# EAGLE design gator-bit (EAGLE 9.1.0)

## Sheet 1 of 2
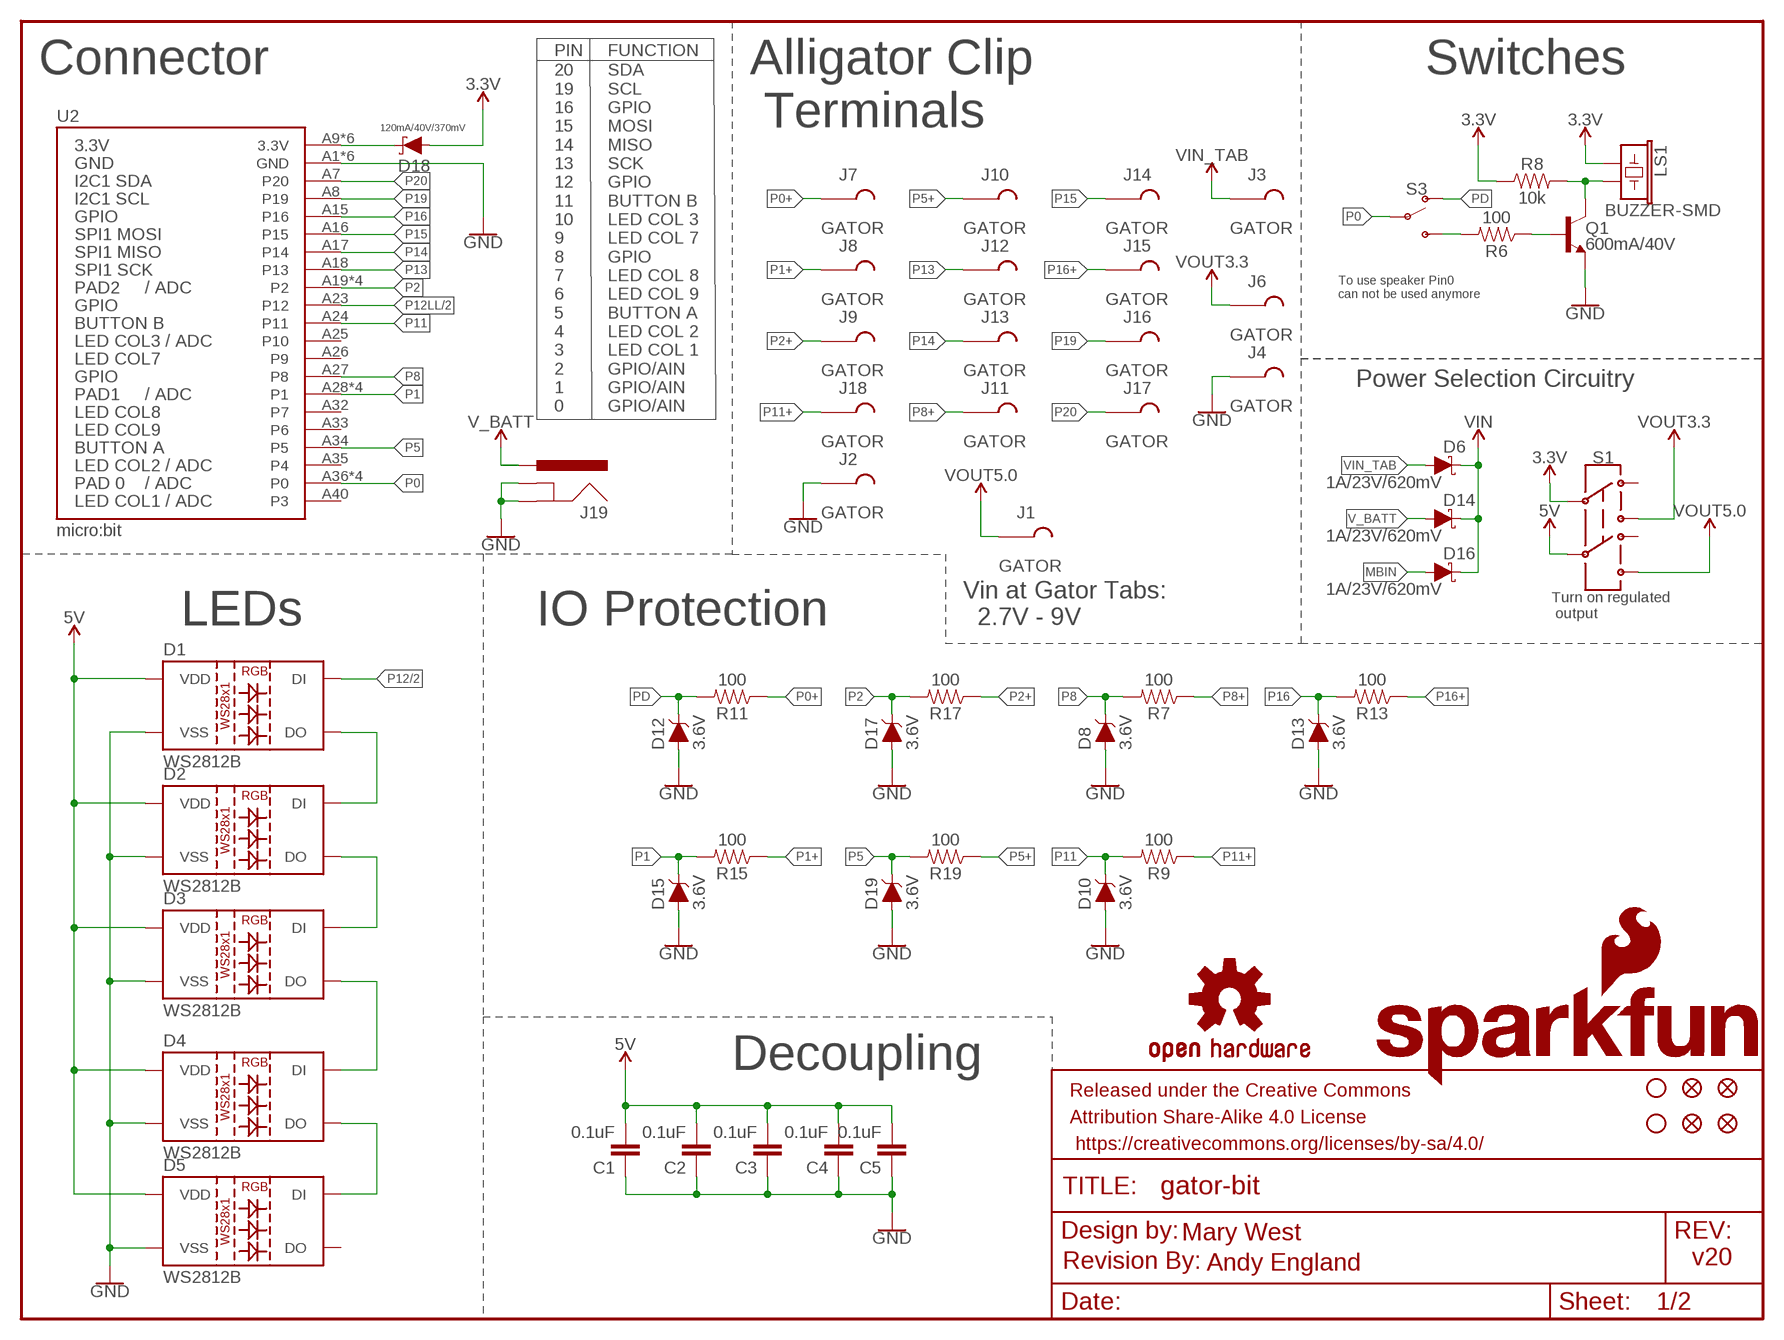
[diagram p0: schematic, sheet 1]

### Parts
C1  0.1uF  0.1UF-0603-25V-(+80/-20%)  [0603]
C2  0.1uF  0.1UF-0603-25V-(+80/-20%)  [0603]
C3  0.1uF  0.1UF-0603-25V-(+80/-20%)  [0603]
C4  0.1uF  0.1UF-0603-25V-(+80/-20%)  [0603]
C5  0.1uF  0.1UF-0603-25V-(+80/-20%)  [0603]
D1  WS2812B  [WS2812B]
D2  WS2812B  [WS2812B]
D3  WS2812B  [WS2812B]
D4  WS2812B  [WS2812B]
D5  WS2812B  [WS2812B]
D6  1A/23V/620mV  DIODE-SCHOTTKY-BAT20J  [SOD-323]
D8  3.6V  DIODE-ZENER-BZT52C3V6S  [SOD-323]
D10  3.6V  DIODE-ZENER-BZT52C3V6S  [SOD-323]
D12  3.6V  DIODE-ZENER-BZT52C3V6S  [SOD-323]
D13  3.6V  DIODE-ZENER-BZT52C3V6S  [SOD-323]
D14  1A/23V/620mV  DIODE-SCHOTTKY-BAT20J  [SOD-323]
D15  3.6V  DIODE-ZENER-BZT52C3V6S  [SOD-323]
D16  1A/23V/620mV  DIODE-SCHOTTKY-BAT20J  [SOD-323]
D17  3.6V  DIODE-ZENER-BZT52C3V6S  [SOD-323]
D18  120mA/40V/370mV  DIODE-SCHOTTKY-RB751S40  [SOD-523]
D19  3.6V  DIODE-ZENER-BZT52C3V6S  [SOD-323]
FD1  FIDUCIAL1X2  [FIDUCIAL-1X2]
FD2  FIDUCIAL1X2  [FIDUCIAL-1X2]
FD3  FIDUCIAL1X2  [FIDUCIAL-1X2]
FD4  FIDUCIAL1X2  [FIDUCIAL-1X2]
FRAME1  FRAME-LETTER  [CREATIVE_COMMONS]
H1  STAND-OFF  [STAND-OFF]
H2  STAND-OFF  [STAND-OFF]
J1  GATOR  [GATOR]
J2  GATOR  [GATOR]
J3  GATOR  [GATOR]
J4  GATOR  [GATOR]
J6  GATOR  [GATOR]
J7  GATOR  [GATOR]
J8  GATOR  [GATOR]
J9  GATOR  [GATOR]
J10  GATOR  [GATOR]
J11  GATOR  [GATOR]
J12  GATOR  [GATOR]
J13  GATOR  [GATOR]
J14  GATOR  [GATOR]
J15  GATOR  [GATOR]
J16  GATOR  [GATOR]
J17  GATOR  [GATOR]
J18  GATOR  [GATOR]
J19  POWER_JACKPTH_LOCK  [POWER_JACK_PTH_LOCK]
LOGO1  SFE_LOGO_NAME_FLAME.3_INCH  [SFE_LOGO_NAME_FLAME_.3]
LOGO2  OSHW-LOGOM  [OSHW-LOGO-M]
LOGO3  REVISION  [REVISION]
LS1  BUZZER-SMD  [BUZZER-CCV]
Q1  600mA/40V  TRANS_NPN-MMBT2222AL  [SOT23-3]
R6  100  100OHM-0603-1/10W-1%  [0603]
R7  100  100OHM-0603-1/10W-1%  [0603]
R8  10k  10KOHM-0603-1/10W-1%  [0603]
R9  100  100OHM-0603-1/10W-1%  [0603]
R11  100  100OHM-0603-1/10W-1%  [0603]
R13  100  100OHM-0603-1/10W-1%  [0603]
R15  100  100OHM-0603-1/10W-1%  [0603]
R17  100  100OHM-0603-1/10W-1%  [0603]
R19  100  100OHM-0603-1/10W-1%  [0603]
S1  SWITCH-DPDT-SMD-AYZ0202  [SWITCH_DPDT_SMD_AYZ0202]
S3  SWITCH-SPDT-SMD-AYZ0202  [SWITCH_DPDT_SMD_AYZ0202]
U2  micro:bit  MICRO:BITLEDS_UP  [MICRO:BIT_RA_PTH]

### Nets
3.3V: D18.A LS1.+ R8.1 S1.2 ; also sheet 2
5V: C1.2 C2.2 C3.2 C4.2 C5.2 D1.1(VDD) D2.1(VDD) D3.1(VDD) D4.1(VDD) D5.1(VDD) S1.5 ; also sheet 2
GND: C1.1 C2.1 C3.1 C4.1 C5.1 D1.3(VSS) D2.3(VSS) D3.3(VSS) D4.3(VSS) D5.3(VSS) D8.A D10.A D12.A D13.A D15.A D17.A D19.A J2.P$1 J2.P$2 J4.P$1 J4.P$2 J19.GND J19.GNDBREAK Q1.2(E) U2.A1(GND) U2.A2(GND) U2.A3(GND) U2.A4(GND) U2.A5(GND) U2.A6(GND) ; also sheet 2
MBIN: D16.A D18.C U2.A9(3.3V) U2.A10(3.3V) U2.A11(3.3V) U2.A12(3.3V) U2.A13(3.3V) U2.A14(3.3V)
N$3: LS1.- Q1.3(C) R8.2
N$4: D1.2(DO) D2.4(DI)
N$5: D2.2(DO) D3.4(DI)
N$6: D3.2(DO) D4.4(DI)
N$7: D4.2(DO) D5.4(DI)
N$20: R6.2 S3.3(S)
N$25: Q1.1(B) R6.1
P0: S3.2(P) U2.A36(P0) U2.A37(P0) U2.A38(P0) U2.A39(P0)
P0+: J7.P$1 J7.P$2 R11.1
P1: D15.C R15.2 U2.A28(P1) U2.A29(P1) U2.A30(P1) U2.A31(P1)
P1+: J8.P$1 J8.P$2 R15.1
P2: D17.C R17.2 U2.A19(P2) U2.A20(P2) U2.A21(P2) U2.A22(P2)
P2+: J9.P$1 J9.P$2 R17.1
P5: D19.C R19.2 U2.A34(P5)
P5+: J10.P$1 J10.P$2 R19.1
P8: D8.C R7.2 U2.A27(P8)
P8+: J11.P$1 J11.P$2 R7.1
P11: D10.C R9.2 U2.A24(P11)
P11+: J18.P$1 J18.P$2 R9.1
P12: D1.4(DI) ; also sheet 2
P12LL: U2.A23(P12) ; also sheet 2
P13: J12.P$1 J12.P$2 U2.A18(P13)
P14: J13.P$1 J13.P$2 U2.A17(P14)
P15: J14.P$1 J14.P$2 U2.A16(P15)
P16: D13.C R13.2 U2.A15(P16)
P16+: J15.P$1 J15.P$2 R13.1
P19: J16.P$1 J16.P$2 U2.A8(P19)
P20: J17.P$1 J17.P$2 U2.A7(P20)
PD: D12.C R11.2 S3.1(O)
V_BATT: D14.A J19.PWR
VIN: D6.C D14.C D16.C ; also sheet 2
VIN_TAB: D6.A J3.P$1 J3.P$2
VOUT3.3: J6.P$1 J6.P$2 S1.3 ; also sheet 2
VOUT5.0: J1.P$1 J1.P$2 S1.6 ; also sheet 2
Unconnected: D5.2(DO) S1.1 S1.4 U2.A25(P10) U2.A26(P9) U2.A32(P7) U2.A33(P6) U2.A35(P4) U2.A40(P3)

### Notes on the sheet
- PIN | FUNCTION
- Connector | Switches
- Alligator Clip
   Terminals
- To use speaker Pin0 
  can not be used anymore
- Power Selection Circuitry
- 20
  19
  16
  15
  14
  13
  12
  11
  10
  9
  8
  7
  6
  5
  4
  3
  2
  1
  0
- SDA
  SCL
  GPIO
  MOSI
  MISO
  SCK
  GPIO
  BUTTON B
  LED COL 3
  LED COL 7
  GPIO
  LED COL 8
  LED COL 9
  BUTTON A
  LED COL 2
  LED COL 1
  GPIO/AIN
  GPIO/AIN
  GPIO/AIN
- Turn on regulated
   output
- LEDs | IO Protection
- Vin at Gator Tabs:
    2.7V - 9V
- Decoupling
- Mary West
- Andy England | v20

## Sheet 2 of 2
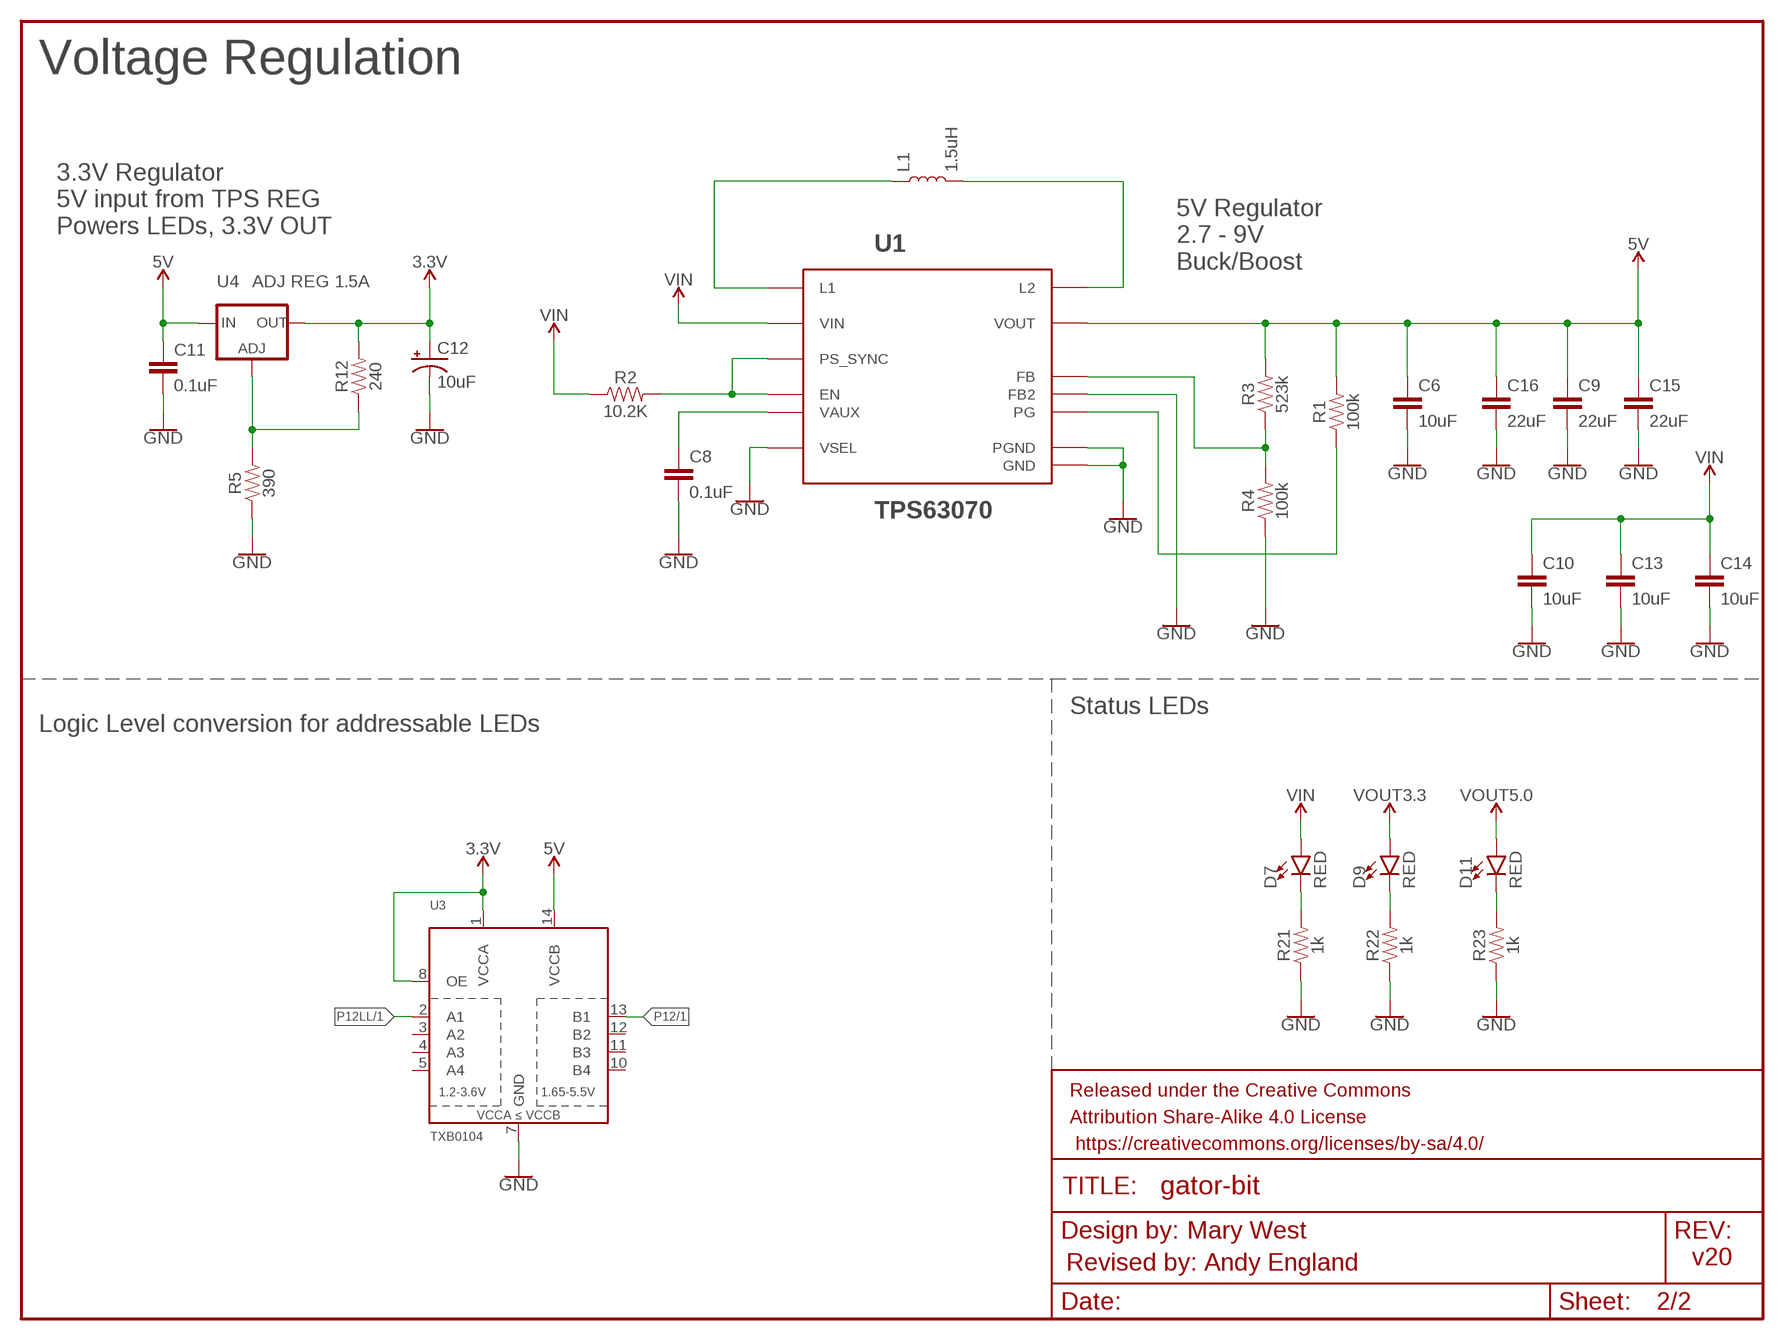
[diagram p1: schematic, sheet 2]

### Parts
C6  10uF  10UF-0603-6.3V-20%  [0603]
C8  0.1uF  0.1UF-0603-25V-(+80/-20%)  [0603]
C9  22uF  22UF-0805-6.3V-20%  [0805]
C10  10uF  10UF-0805-10V-10%  [0805]
C11  0.1uF  0.1UF-0603-25V-(+80/-20%)  [0603]
C12  10uF  10UF-POLAR-EIA3216-16V-10%(TANT)  [EIA3216]
C13  10uF  10UF-0805-10V-10%  [0805]
C14  10uF  10UF-0603-6.3V-20%  [0603]
C15  22uF  22UF-0805-6.3V-20%  [0805]
C16  22uF  22UF-0805-6.3V-20%  [0805]
D7  RED  LED-RED0603  [LED-0603]
D9  RED  LED-RED0603  [LED-0603]
D11  RED  LED-RED0603  [LED-0603]
FRAME3  FRAME-LETTER  [CREATIVE_COMMONS]
L1  1.5uH  INDUCTOR-XFL40201.5UH  [XFL4020]
R1  100k  100KOHM-0603-1/10W-1%  [0603]
R2  10.2K  10.2KOHM  [0603]
R3  523k  523KOHMOHMS-0603-1/10W-1%  [0603]
R4  100k  100KOHM-0603-1/10W-1%  [0603]
R5  390  390OHM-0603-1/10W-1%  [0603]
R12  240  240OHM-0603-1/10W-1%  [0603]
R21  1k  1KOHM-0603-1/10W-1%  [0603]
R22  1k  1KOHM-0603-1/10W-1%  [0603]
R23  1k  1KOHM-0603-1/10W-1%  [0603]
U1  TPS63070  TPS63070RNM  [TPS63070RNM]
U3  TXB0104  TXB0104PWR  [TSSOP14]
U4  ADJ REG 1.5A  GATORBIT_LM317  [SOT223]

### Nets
3.3V: C12.+ R12.2 U3.1(VCCA) U3.8(OE) U4.2(OUT) U4.4(OUT) ; also sheet 1
5V: C6.1 C9.1 C11.1 C15.1 C16.1 R1.2 R3.2 U1.P$7(VOUT) U3.14(VCCB) U4.3(IN) ; also sheet 1
GND: C6.2 C8.2 C9.2 C10.2 C11.2 C12.- C13.2 C14.2 C15.2 C16.2 R4.1 R5.1 R21.1 R22.1 R23.1 U1.P$4(GND) U1.P$6(FB2) U1.P$10(PGND) U1.P$15(VSEL) U3.7(GND) ; also sheet 1
N$2: L1.P$1 U1.P$11(L1)
N$8: L1.P$2 U1.P$9(L2)
N$9: D7.C R21.2
N$11: R3.1 R4.2 U1.P$5(FB)
N$12: C8.1 U1.P$3(VAUX)
N$13: R2.2 U1.P$1(PS_SYNC) U1.P$14(EN)
N$14: R1.1 U1.P$2(PG)
N$16: R5.2 R12.1 U4.1(ADJ)
N$23: D9.C R22.2
N$24: D11.C R23.2
P12: U3.13(B1) ; also sheet 1
P12LL: U3.2(A1) ; also sheet 1
VIN: C10.1 C13.1 C14.1 D7.A R2.1 U1.P$12(VIN) ; also sheet 1
VOUT3.3: D9.A ; also sheet 1
VOUT5.0: D11.A ; also sheet 1
Unconnected: U3.3(A2) U3.4(A3) U3.5(A4) U3.10(B4) U3.11(B3) U3.12(B2)

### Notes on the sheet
- Voltage Regulation
- 3.3V Regulator
  5V input from TPS REG
  Powers LEDs, 3.3V OUT
- 5V Regulator
  2.7 - 9V
  Buck/Boost
- Status LEDs
- Logic Level conversion for addressable LEDs
- Mary West
- Revised by: Andy England | v20

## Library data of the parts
C1-C5 C8 C11 = SparkFun-Capacitors:0.1UF: 0.1µF ceramic capacitors; PROD_ID: CAP-00810
C6 C14 = SparkFun-Capacitors:10UF: 10.0µF ceramic capacitors; PROD_ID: CAP-11015
C9 C15 C16 = SparkFun-Capacitors:22UF: 22µF ceramic capacitors; PROD_ID: CAP-08402
C10 C13 = SparkFun-Capacitors:10UF: 10.0µF ceramic capacitors; PROD_ID: CAP-11330
C12 = SparkFun-Capacitors:10UF-POLAR: 10.0µF polarized capacitors; PROD_ID: CAP-00811
D1-D5 = SparkFun-LED:WS2812B: WS2812B SMD addressable RGB LED 5x5mm SMD LED with built-in controller IC. Color: Red/Green/Blue mC Rating: RGB: 390, 660, 180 mcd Forward Voltage: RGB: 2.0, 3.0, 3.0 V Packages:WS2812B SparkFun Products: Blynk Board - ESP8266; PROD_ID: DIO-12503
D6 D14 D16 = SparkFun-DiscreteSemi:DIODE-SCHOTTKY: Schottky diode; PROD_ID: DIO-11623
D7 D9 D11 = SparkFun-LED:LED-RED: Red SMD LED; PROD_ID: DIO-00819
D8 D10 D12 D13 D15 D17 D19 = SparkFun-DiscreteSemi:DIODE-ZENER: Zener Diode; PROD_ID: DIO-08199
D18 = SparkFun-DiscreteSemi:DIODE-SCHOTTKY: Schottky diode; PROD_ID: DIO-11018
FD1-FD4 = SparkFun-Aesthetics:FIDUCIAL: Fiducial Alignment Points
FRAME1 FRAME3 = SparkFun-Aesthetics:FRAME-LETTER: Schematic Frame - Letter
H1 H2 = SparkFun-Hardware:STAND-OFF: Stand Off
J1-J4 J6-J18 = TAB:GATOR
J19 = SparkFun-Connectors:POWER_JACK: Power Jack Connector This is the standard 5.5mm barrel jack for power. The PTH is the most common, proven, reliable, footprint. The Slot footprint only works if the mill layer is transmitted to the PCB fab house so be warned. Here are the connectors we sell at SparkFun: DC Barrel Power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; PROD_ID: CONN-08197; SF_ID: PRT-00119
L1 = SparkFun-Coils:INDUCTOR-XFL4020; PROD_ID: INDUC-13855
LOGO1 = SparkFun-Aesthetics:SFE_LOGO_NAME_FLAME: SparkFun Font Logo w/ Flame
LOGO2 = SparkFun-Aesthetics:OSHW-LOGO: Open-Source Hardware (OSHW) Logo
LOGO3 = SparkFun-Aesthetics:REVISION: "Revision By" Text
LS1 = SparkFun-Electromechanical:BUZZER: Buzzer; PROD_ID: COMP-08568
Q1 = SparkFun-DiscreteSemi:TRANS_NPN: NPN transistor Current controlled devices typically used to amplify current or used as a switch. BC547 - COM-08928 (TO-92 45V 100mA) (1.Collector 2.Base 3.Emitter) 2N3904 - COM-00521 (TO-92 40V 200mA) (1.Emitter 2.Base 3.Collector) P2N2222A - COM-12852 (TO-92 40V 600mA) (1.Collector 2.Base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; PROD_ID: TRANS-08049
R1 R4 = SparkFun-Resistors:100KOHM: 100kΩ resistor; PROD_ID: RES-07828
R2 = SparkFun-Resistors:10.2KOHM: https://www.digikey.com/product-detail/en/yageo/RC0603FR-0710K2L/311-10.2KHRTR-ND/726883; PROD_ID: RES-13856
R3 = SparkFun-Resistors:523KOHM; PROD_ID: RES-13864
R5 = SparkFun-Resistors:390OHM: 390Ω resistor; PROD_ID: RES-07864
R6 R7 R9 R11 R13 R15 R17 R19 = SparkFun-Resistors:100OHM: 100Ω resistor; PROD_ID: RES-07863
R8 = SparkFun-Resistors:10KOHM: 10kΩ resistor; PROD_ID: RES-00824
R12 = SparkFun-Resistors:240OHM: 240Ω resistor; PROD_ID: RES-07849
R21-R23 = SparkFun-Resistors:1KOHM: 1kΩ resistor; PROD_ID: RES-07856
S1 = SparkFun-Switches:SWITCH-DPDT: Double-Pole, Double-Throw (DPDT) Switch Double-pole, double-throw switches. Variant Overview PTH-GPI-152-3013 Used on SparkFun Geiger Counter SMD-AY0202 Surface Mount DPDT Switch (COM-00597) Used on e.g. LilyPad Arduino USB - ATmega32U4 Board; PROD_ID: SWCH-08179; SF_SKU: COM-00597
S3 = SparkFun-Switches:SWITCH-SPDT: Single Pole, Double Throw (SPDT) Switch Single-pole, double-throw (SPDT) switch. Variant Overview SMD-AYZ0202 Surface Mount DPDT Switch (COM-00597) Used on e.g. LilyPad Arduino USB - ATmega32U4 Board PTH-11.6X4.0MM SPDT Mini Power Switch (COM-00102) Used on e.g. SparkFun Simon Says - Through-Hole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; PROD_ID: SWCH-08179; SF_ID: COM-00597
U1 = SparkFun-IC-Power:TPS63070RNM: The TPS6307x is a high efficiency, low quiescent current buck-boost converter suitable for applications where the input voltage can be higher or lower than the output voltage. Output currents can go as high as 2 A in boost mode and in buck mode. The buck-boost converter is based on a fixed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; PROD_ID: IC-13858
U2 = Micro_Bit_Parts:MICRO:BIT: BBC MICRO_BIT with 5x5 LED array facing the direction noted in the variant. "UP" means away from the host board, "Down" means facing towards the host board.; PROD_ID: CONN-13452
U3 = SparkFun-IC-Comms:TXB0104PWR: 4-Bit Bi-Directional Level Shifter 1.2V-3.6V (VCCA) to 1.65V-5.5V (VCCB) bi-directional level shifter with auto direction sensing. Max data rate - VCCA 1.8V: 20Mbps (50ns), VCCA 3.3V: 100Mbps (10ns) Digikey: 296-21929-1-ND (TSSOP) Datasheet SparkFun Products SparkFun Cellular Shield - MG2639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; PROD_ID: IC-13929
U4 = SparkFun-IC-Power:GATORBIT_LM317; PROD_ID: VREG-12029

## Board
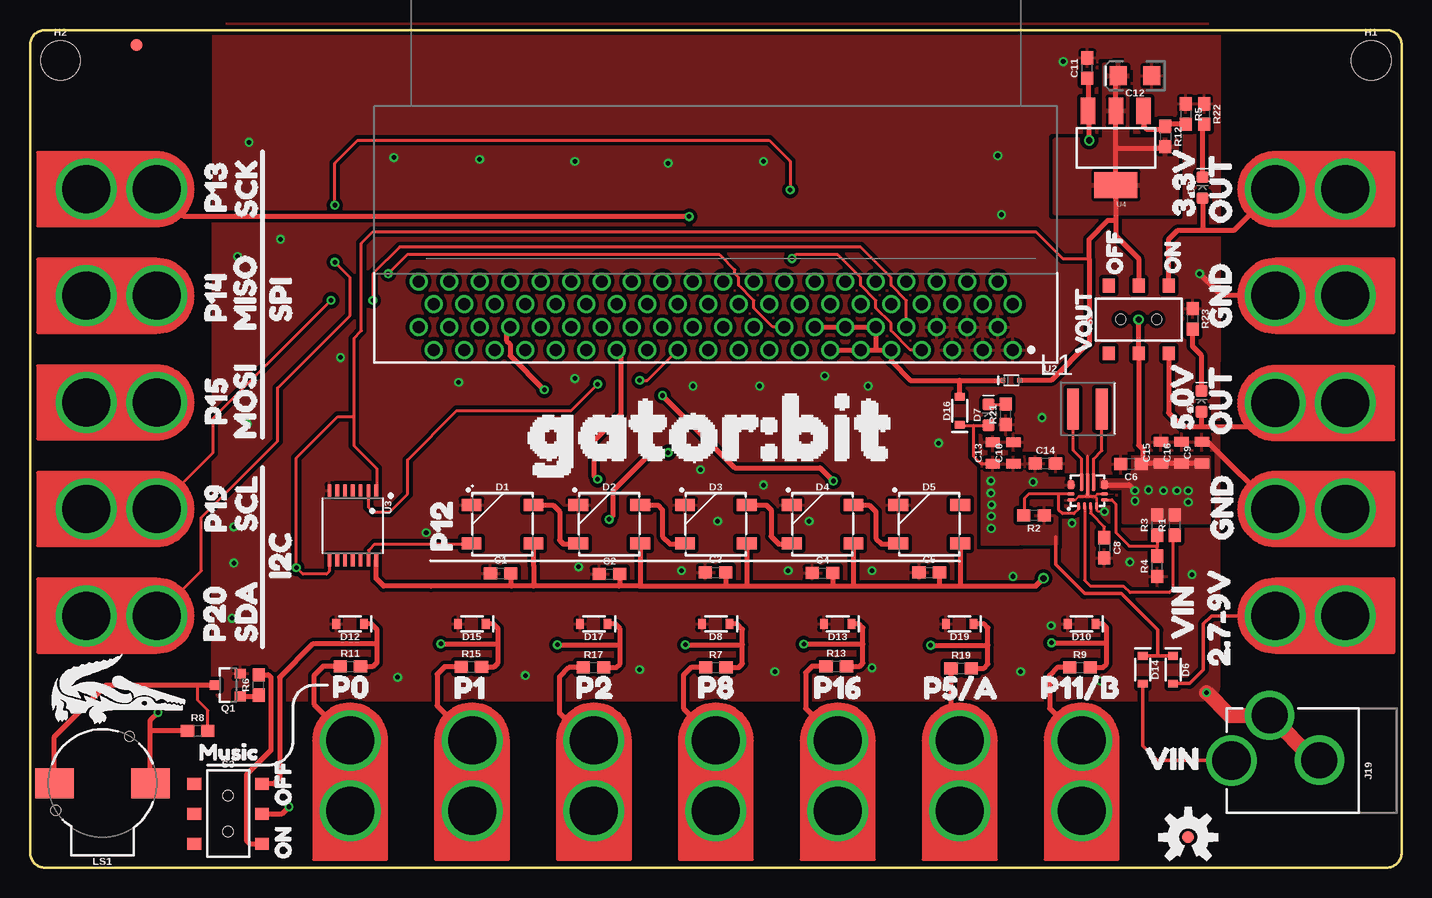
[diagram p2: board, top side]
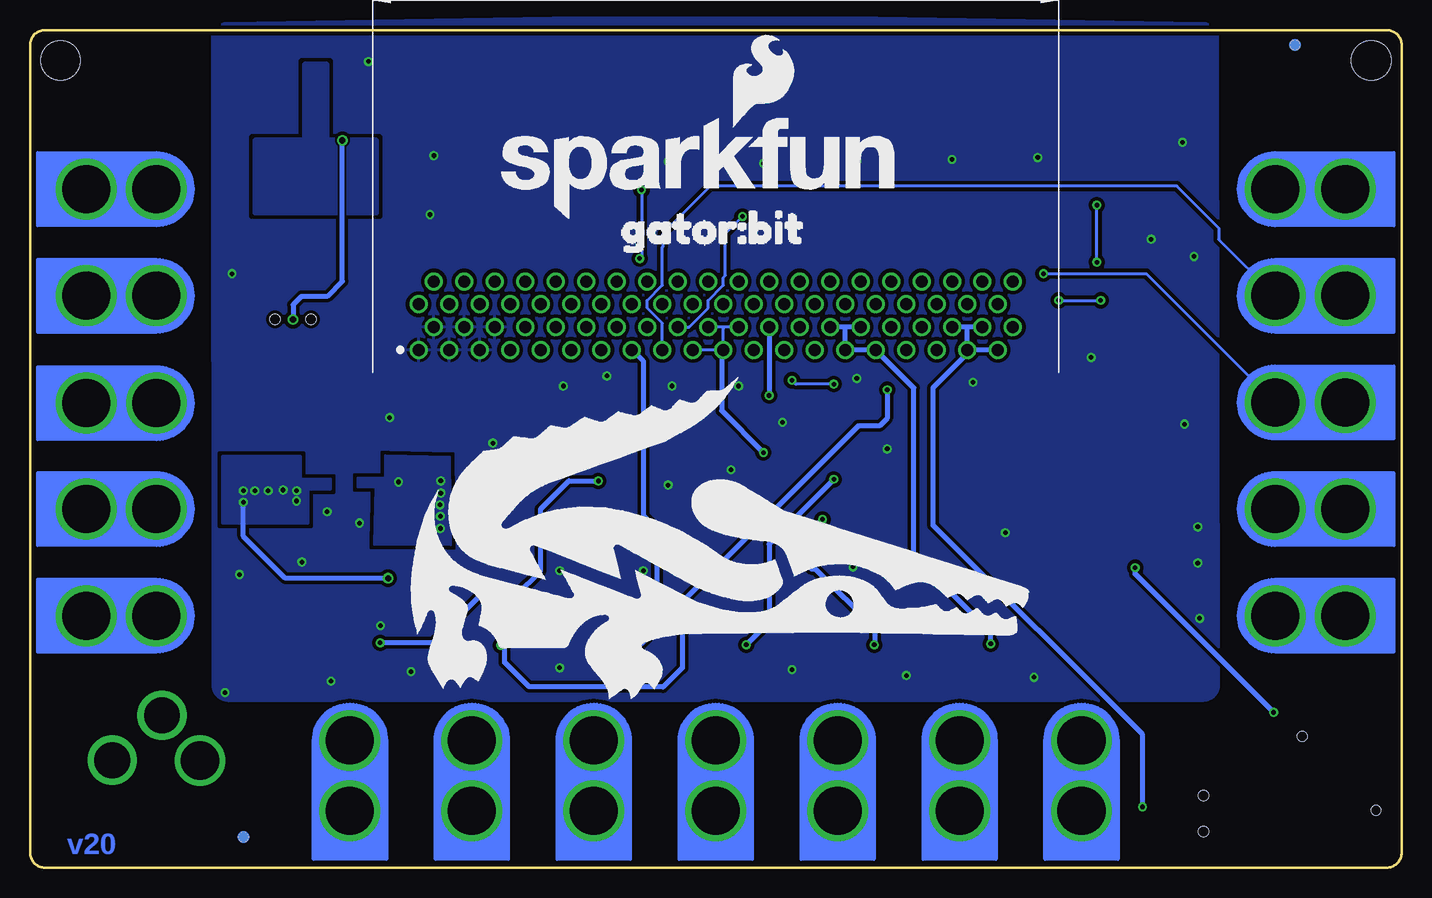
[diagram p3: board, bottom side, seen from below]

Size 114.3 x 69.85 mm. Coordinates in mm from the lower left corner, seen from the top.
Outline: 0,68.58 0,1.27 arc90 1.27,0 113.03,0 arc90 114.3,1.27 114.3,68.58 arc90 113.03,69.85 1.27,69.85 arc90 0,68.58
Copper layers (1*16): Top 0.035mm / dielectric 1.5mm / Bottom 0.035mm
Design rules "SparkFun-2-layer-TIGHT": minimum track width 7mil, minimum drill 15mil, track to track 7mil, track to pad 7mil, pad to pad 7mil, via to via 7mil, smd to smd 7mil, copper to edge 7mil, drill to drill 7mil, minimum pad ring 7mil, minimum via ring 7mil, stop-mask expansion 4mil, vias tented up to drill 25mil, thermal gap 10mil

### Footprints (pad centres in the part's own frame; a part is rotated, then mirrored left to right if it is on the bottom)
0603 = smd 1.1 x 1: 1 -0.85,0; 2 0.85,0
0805 = smd 0.8 x 1.2: 1 -0.9,0; 2 0.9,0
EIA3216 = smd 1.4 x 1.6: + 1.4,0; - -1.4,0
WS2812B = smd 1.651 x 1: 1 2.577,-1.6; 2 2.577,1.6; 3 -2.577,1.6; 4 -2.577,-1.6
SOD-323 = smd 0.63 x 0.83: A 1.15,0; C -1.15,0
LED-0603 = smd 1 x 1: A -0.877,0; C 0.877,0
SOD-523 = smd 0.4 x 0.4: A -0.7,0; C 0.7,0
FIDUCIAL-1X2 = smd 1 x 1: 1 0,0
STAND-OFF = hole 3.302: 0,0
GATOR = drill 4 pad 5.08: P$1 0,-6.096; P$2 0,-0.254
POWER_JACK_PTH_LOCK = drill 2.997 pad 4.115: GND 0.025,6.557; GNDBREAK 3.762,10.7 | drill 3.2 pad 4.115: PWR 0,13.878
XFL4020 = smd 0.98 x 3.4: P$1 1,1.8; P$2 3.4,1.8
BUZZER-CCV = smd 3.2 x 2.5: + 4,0; - -4,0 | hole 0.8: -3.9,-2.25; 2.25,3.9
SOT23-3 = smd 0.8 x 0.9: 1 -0.95,-1; 2 0.95,-1; 3 0,1.1
SWITCH_DPDT_SMD_AYZ0202 = smd 1 x 1.15: 1 -2.5,2.825; 2 0,2.825; 3 2.5,2.825; 4 -2.5,-2.825; 5 0,-2.825; 6 2.5,-2.825 | hole 0.85: 1.5,0; -1.5,0
TPS63070RNM = smd 0.6 x 0.25: P$1 0,2.145; P$2 0,1.645; P$3 0,1.145; P$4 0,0.645 | smd 0.25 x 0.6: P$5 0.5,-0.005; P$6 1,-0.005; P$14 1,2.795; P$15 0.5,2.795 | smd 0.75 x 0.6: P$7 1.757,0.006; P$12 1.768,2.794 | smd 1.45 x 0.35: P$9 1.988,0.895; P$11 1.988,1.895 | smd 1.8 x 0.35: P$10 1.812,1.395
MICRO:BIT_RA_PTH = drill 1: A1 -24.765,7.62; A2 -23.495,5.72; A3 -22.225,7.62; A4 -20.955,5.72; A5 -19.685,7.62; A6 -18.415,5.72; A7 -17.145,7.62; A8 -15.875,5.72; A9 -14.605,7.62; A10 -13.335,5.72; A11 -12.065,7.62; A12 -10.795,5.72; A13 -9.525,7.62; A14 -8.255,5.72; A15 -6.985,7.62; A16 -5.715,5.72; A17 -4.445,7.62; A18 -3.175,5.72; A19 -1.905,7.62; A20 -0.635,5.72; A21 0.635,7.62; A22 1.905,5.72; A23 3.175,7.62; A24 4.445,5.72; A25 5.715,7.62; A26 6.985,5.72; A27 8.255,7.62; A28 9.525,5.72; A29 10.795,7.62; A30 12.065,5.72; A31 13.335,7.62; A32 14.605,5.72; A33 15.875,7.62; A34 17.145,5.72; A35 18.415,7.62; A36 19.685,5.72; A37 20.955,7.62; A38 22.225,5.72; A39 23.495,7.62; A40 24.765,5.72; B1 -24.765,3.82; B2 -23.495,1.92; B3 -22.225,3.82; B4 -20.955,1.92; B5 -19.685,3.82; B6 -18.415,1.92; B7 -17.145,3.82; B8 -15.875,1.92; B9 -14.605,3.82; B10 -13.335,1.92; B11 -12.065,3.82; B12 -10.795,1.92; B13 -9.525,3.82; B14 -8.255,1.92; B15 -6.985,3.82; B16 -5.715,1.92; B17 -4.445,3.82; B18 -3.175,1.92; B19 -1.905,3.82; B20 -0.635,1.92; B21 0.635,3.82; B22 1.905,1.92; B23 3.175,3.82; B24 4.445,1.92; B25 5.715,3.82; B26 6.985,1.92; B27 8.255,3.82; B28 9.525,1.92; B29 10.795,3.82; B30 12.065,1.92; B31 13.335,3.82; B32 14.605,1.92; B33 15.875,3.82; B34 17.145,1.92; B35 18.415,3.82; B36 19.685,1.92; B37 20.955,3.82; B38 22.225,1.92; B39 23.495,3.82; B40 24.765,1.92
TSSOP14 = smd 0.305 x 0.991: 1 -1.95,-2.918; 2 -1.3,-2.918; 3 -0.65,-2.918; 4 0,-2.918; 5 0.65,-2.918; 6 1.3,-2.918; 7 1.95,-2.918; 8 1.95,2.918; 9 1.3,2.918; 10 0.65,2.918; 11 0,2.918; 12 -0.65,2.918; 13 -1.3,2.918; 14 -1.95,2.918
SOT223 = smd 1.219 x 2.235: 1 -2.311,-3.099; 2 0,-3.099; 3 2.311,-3.099 | smd 3.6 x 2.2: 4 0,3.099

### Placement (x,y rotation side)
C1  39.22,24.56 0 top
C2  48.29,24.49 0 top
C3  57.13,24.62 0 top
C4  66.05,24.56 0 top
C5  74.94,24.62 0 top
C6  91.76,33.66 180 top
C8  89.54,26.67 270 top
C9  97.65,34.61 90 top
C10  81.95,34.58 90 top
C11  88.11,66.67 90 top
C12  92.08,66.04 180 top
C13  80.23,34.58 90 top
C14  84.61,33.72 0 top
C15  94.25,34.61 90 top
C16  95.96,34.61 90 top
D1  39.38,28.64 0 top
D2  48.27,28.64 0 top
D3  57.16,28.64 0 top
D4  66.05,28.64 0 top
D5  74.94,28.64 0 top
D6  95.25,16.51 270 top
D7  79.88,37.76 90 top
D8  57.15,20.32 180 top
D9  97.71,56.71 90 top
D10  87.63,20.32 180 top
D11  97.64,38.89 90 top
D12  26.67,20.32 180 top
D13  67.31,20.32 180 top
D14  92.71,16.51 270 top
D15  36.83,20.32 180 top
D16  77.47,38.1 90 top
D17  46.99,20.32 180 top
D18  81.79,40.64 180 top
D19  77.47,20.32 180 top
FD1  96.52,2.54 0 bottom
FD2  8.89,68.58 0 top
FD3  96.52,2.54 0 top
FD4  8.89,68.58 0 bottom
FRAME1  not placed on the board
FRAME3  not placed on the board
H1  111.76,67.31 0 top
H2  2.54,67.31 0 top
J1  103.51,38.73 90 top
J2  103.51,47.69 90 top
J3  103.51,21.02 90 top
J4  103.51,29.91 90 top
J6  103.51,56.58 90 top
J7  26.68,10.86 0 top
J8  36.84,10.86 0 top
J9  47,10.86 0 top
J10  77.48,10.86 0 top
J11  57.16,10.86 0 top
J12  10.8,56.58 270 top
J13  10.8,47.69 270 top
J14  10.8,38.8 270 top
J15  67.32,10.86 0 top
J16  10.8,29.91 270 top
J17  10.8,21.02 270 top
J18  87.64,10.86 0 top
J19  114,8.94 90 top
L1  85.92,36.46 0 top
LOGO1  75.57,53.98 0 bottom
LOGO2  96.52,2.54 0 top
LOGO3  not placed on the board
LS1  6.04,7.04 0 top
Q1  16.51,15.24 90 top
R1  95.42,28.57 90 top
R2  83.66,29.37 180 top
R3  93.94,28.57 90 top
R4  93.94,25.13 90 top
R5  96.32,62.84 270 top
R6  19.05,15.24 90 top
R7  57.15,16.69 0 top
R8  13.97,11.43 0 top
R9  87.5,16.69 0 top
R11  26.7,16.79 0 top
R12  94.62,60.96 270 top
R13  67.19,16.8 0 top
R15  36.78,16.76 0 top
R17  46.96,16.69 0 top
R19  77.6,16.64 0 top
R21  81.32,37.81 90 top
R22  97.84,62.84 270 top
R23  96.88,45.77 270 top
S1  92.39,45.72 0 top
S3  16.52,4.5 270 top
U1  89.54,30.16 90 top
U2  57.15,50.8 180 top
U3  26.9,28.52 180 top
U4  90.49,60.01 180 top
U$1  [2#7#9V21]  99.06,15.24 90 top
U$2  [3#3V25]  96.14,52.7 90 top
U$3  [5#0V23]  96.01,34.92 90 top
U$4  [ORDERING_INSTRUCTIONS]  not placed on the board
U$5  [GATOR#BIT26]  36.88,36.63 0 top
U$6  [GATOR#BIT32]  67.31,53.34 0 bottom
U$7  [GND22]  99.31,25.78 90 top
U$8  [GND22]  99.19,43.43 90 top
U$9  [I2C7]  20.83,22.48 90 top
U$10  [MISO5]  17.91,43.18 90 top
U$11  [MOSI4]  17.91,34.16 90 top
U$12  [MUSIC28]  12.95,9.65 0 top
U$13  [OFF29]  21.08,4.06 90 top
U$14  [ON30]  21.08,-0.38 90 top
U$15  [OUT24]  99.19,34.54 90 top
U$16  [OUT24]  99.19,52.2 90 top
U$17  [P5#A18]  72.85,14.99 0 top
U$18  [P11#B19]  82.6,15.04 0 top
U$19  [P013]  23.57,15.09 0 top
U$20  [P114]  33.71,15.01 0 top
U$21  [P130]  15.47,53.04 90 top
U$22  [P199]  15.47,26.34 90 top
U$23  [P208]  15.37,17.25 90 top
U$24  [P215]  43.87,15.04 0 top
U$25  [P816]  54.03,15.06 0 top
U$26  [P1227]  34.29,24.77 90 top
U$27  [P1411]  15.47,43.89 90 top
U$28  [P1510]  15.49,35.33 90 top
U$29  [P1617]  63.68,15.04 0 top
U$30  [SCK1]  18.01,52.65 90 top
U$31  [SCL2]  18.01,26.47 90 top
U$32  [SDA3]  18.01,17.22 90 top
U$33  [SPI6]  20.88,43.97 90 top
U$34  [VIN20]  96.04,17.48 90 top
U$35  [VOUT31]  87.78,41.76 90 top
U$36  [OFF29]  90.37,48.34 90 top
U$37  [ON30]  95.2,48.41 90 top
U$39  [VIN20]  91.39,9.09 0 top

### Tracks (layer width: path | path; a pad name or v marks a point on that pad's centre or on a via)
3.3V  (via drill 0.38)
  Top 0.254: 88.27,50.8 86.04,50.8 83.82,53.02 28.57,53.02 27.62,52.07 27.62,44.77 26.99,44.13 26.99,37.72 | 26.99,37.72 26.99,35.19 28.88,33.3 28.88,31.47 U3.1 | U3.8 24.95,24.72 24.71,24.49 22.73,24.49 v22.2,25.02 22.2,34.16 25.65,37.62 26.89,37.62 26.99,37.72
  Top 0.406: 90.49,53.98 U4.4 90.49,60.01 | 90.49,53.98 90.49,52.7 92.39,50.8 S1.2 | 90.49,53.98 89.85,53.98 88.27,52.39 88.27,50.8 88.27,43.81 85.09,40.64 D18.A | C12.+ 90.49,65.85 U4.2 90.49,60.01 | 90.49,60.01 94.51,60.01 R12.2 | v10.67,12.95 10.04,12.32 10.04,11.43 | LS1.+ 10.04,11.43 | R8.1 10.04,11.43
  Bottom 0.406: v10.67,12.95 22.2,24.49 v22.2,25.02
  pour Top (isolate 0.305): 89.54,66.99 89.54,60.64 85.41,60.64 85.41,54.61 95.57,54.61 95.57,60.64 91.44,60.64 91.44,66.99
5V  (via drill 0.38, 0.51)
  Top 0.406: C11.1 88.18,65.75 U4.3 88.27,63.02 v88.27,60.64 | 50.8,23.5 58.1,23.5 | 58.1,23.5 59.69,23.5 | 59.69,23.5 66.99,23.5 | 66.99,23.5 68.58,23.5 | 68.58,23.5 75.88,23.5 | 75.88,23.5 77.47,23.5 | 77.47,23.5 83.82,23.5 v84.45,24.13 | D1.1 41.95,25.18 41.96,25.18 41.96,23.5 | D2.1 50.84,23.54 50.8,23.5 | 58.1,23.5 57.98,23.62 C3.2 | D3.1 59.73,23.54 59.69,23.5 | C4.2 66.89,23.59 66.99,23.5 | D4.1 68.62,23.54 68.58,23.5 | C5.2 75.78,23.59 75.88,23.5 | D5.1 77.51,23.54 77.47,23.5 | C9.1 C16.1 C15.1 92.66,33.71 C6.1 92.71,33.76 92.71,34.92 92.39,35.24 S1.5 92.39,45.69 v92.38,45.71 | U1.P$7 91.59,31.92 v92.08,31.43 | 50.8,23.5 49.1,23.5 | 49.1,23.5 41.96,23.5 | 41.96,23.5 40.13,23.5 | 40.13,23.5 33.4,23.5 29.46,23.5 28.85,24.11 U3.14 | C1.2 40.07,23.55 40.13,23.5 | C2.2 49.14,23.54 49.1,23.5
  Bottom 0.406: v84.45,24.13 93.03,24.13 96.52,27.62 v96.52,30.48 | v88.27,60.64 88.27,48.9 89.53,47.62 91.69,47.62 92.38,46.93 v92.38,45.71
  other vias: 95.57,31.43 94.46,31.43 93.21,31.5 96.52,31.43 92.09,30.58
  pour Top (isolate 0.305, no thermals): 89.22,32.38 91.76,32.38 91.76,34.29 98.27,34.29 98.27,28.73 91.12,28.73 91.12,31.59 89.22,31.59
  pour Bottom: 91.12,28.73 91.12,31.59 89.22,31.59 89.22,32.38 91.76,32.38 91.76,34.29 98.27,34.29 98.27,28.73
GND  (via drill 0.38)
  Top 0.203: 88.73,30.93 88.96,31.16 U1.P$6 | 88.73,30.93 88.89,30.78 U1.P$4 88.89,29.86 88.9,29.84 88.9,29.81 89.02,29.69 v89.53,29.69 | U1.P$15 87.03,30.66 87.05,30.68 87.12,30.68 87.38,30.94 88.73,30.94 88.73,30.93
  Top 0.254: U1.P$10 88.14,34.32
  Top 0.406: J2.P$1 J2.P$2 99.32,47.69 97.63,49.37 | J4.P$1 J4.P$2 98.16,35.51 C9.2
  Top 1.27: v98.04,14.61 99.95,12.7 J19.GNDBREAK 107.04,8.96 J19.GND
  other vias: 97.47,49.53 16.99,25.4 16.83,20.8 30.64,15.88 41.28,16.03 50.8,16.51 62.07,16.35 57.31,28.89 16.99,28.42 18.26,60.48 17.3,50.96 20.87,52.41 42.86,34.92 37.47,59.05 45.4,58.9 53.18,58.74 69.85,40.16 61.12,58.9 45.4,40.8 51.59,37.15 61.12,31.91 84.33,37.53 18.1,36.99 80.65,59.37 86.11,67.21 80.96,54.45 86.84,28.73 75.72,35.4 81.92,24.29 91.65,25.49 70.17,16.67 82.55,16.35 55.88,33.18 64.93,28.89 30.32,59.21 25.88,42.55 60.8,40.16 55.25,40.16 85.09,20.18 96.84,24.45 89.22,15.56 35.72,40.48 66.23,41.01 70.17,24.77 63.18,24.77 54.29,24.77 45.72,25.08 33.02,27.94
  pour Top (isolate 0.305, rank 2): 15.24,15.24 15.3,69.12 arc-90 16.57,70.39 97.85,70.39 arc-90 99.12,69.12 99.06,15.24 arc-90 97.79,13.97 16.51,13.97 arc-90
  pour Bottom (isolate 0.305, rank 2): 15.24,15.24 15.3,69.12 arc-90 16.57,70.39 arc-3 97.85,70.39 arc-90 99.12,69.12 99.06,15.24 arc-90 97.79,13.97 16.51,13.97 arc-90
MBIN
  Top 0.406: U2.A13 U2.A11 70.48,43.18 | 70.48,43.18 U2.A9 71.75,42.23 73.34,40.64 77.47,40.64 | U2.A14 U2.A12 U2.A10 70.48,43.18 | 77.47,40.64 D18.C | D16.A 77.47,40.64
N$2
  Top 0.254: U1.P$11 87.64,34.09 86.93,34.8 86.94,34.81 86.94,38.24 L1.P$1
N$3
  Top 0.254: R8.2 14.82,13.12 13.97,13.97 13.97,15.24
  Top 0.406: LS1.- 2.04,10.93 6.35,15.24 13.97,15.24 Q1.3
N$4
  Top 0.406: D1.2 43.58,30.23 44.13,29.69 44.13,27.3 44.45,26.99 46.04,26.99 46.2,26.83 45.89,26.83 D2.4
N$5
  Top 0.406: D2.2 52.31,30.23 52.7,29.84 52.7,27.62 53.34,26.99 54.53,26.99 D3.4
N$6
  Top 0.406: D3.2 61.36,30.23 61.75,29.84 61.75,27.62 62.39,26.99 63.42,26.99 D4.4
N$7
  Top 0.406: D4.2 69.94,30.23 70.48,29.69 70.48,27.46 70.96,26.99 72.31,26.99 D5.4
N$8
  Top 0.254: U1.P$9 88.64,34.09 89.33,34.78 89.33,38.25 L1.P$2
N$9
  Top 0.254: D7.C 81.31,38.64 R21.2
N$11
  Top 0.254: U1.P$5 90.15,30.66 90.49,30.32 90.49,27.94 91.6,26.83 93.87,26.83 93.95,26.75 | R3.1 93.95,27.71 93.95,26.75 | R4.2 93.94,26.73 93.95,26.75
N$12
  Top 0.254: U1.P$3 88.39,29.56 89.53,28.42 C8.1
N$13
  Top 0.254: U1.P$1 87.39,29.92 87,29.53 86.04,29.53 85.72,29.84 85.72,31.16 | U1.P$14 85.72,31.16 | 85.72,31.16 83.23,31.16 82.87,30.8 82.87,29.43 R2.2
N$14
  Top 0.254: U1.P$2 87.89,23.96 88.36,23.5 91.12,23.5 91.68,22.94 94.94,22.94 95.26,23.25 95.26,27.57 R1.1
N$16
  Top 0.406: U4.1 92.8,61.82 93.03,61.59 94.4,61.59 R12.1 94.8,61.99 R5.2
N$20
  Top 0.406: R6.2 19.85,16.09 20.07,15.88 20.07,9.78 18.03,7.75 18.03,2.29 18.32,2 S3.3
N$22
  pour Bottom: 89.54,66.99 91.44,66.99 91.44,60.64 95.57,60.64 95.57,54.61 85.41,54.61 85.41,60.64 89.54,60.64
N$23
  Top 0.406: D9.C 97.71,61.86 R22.2
N$24
  Top 0.406: D11.C 97.64,42.7 96.88,43.46 R23.2
N$25
  Top 0.406: Q1.1 18.95,14.29 R6.1
P0  (via drill 0.38)
  Top 0.406: S3.2 21.02,4.5 v21.59,5.08
  Bottom 0.406: U2.A38 36.2,45.08 | 36.2,45.08 U2.A36 | U2.A37 36.2,45.08 | U2.A39 U2.A37 | U2.A37 36.2,42.86 39.05,40.01 39.05,28.57 21.59,11.11 v21.59,5.08
P0+
  Top 0.406: J7.P$1 J7.P$2 23.65,13.63 23.65,16 24.43,16.79 R11.1
P1  (via drill 0.38)
  Top 0.406: R15.2 38.68,16.76 39,17.08 39,18.67 | v34.24,18.67 39,18.67 | 39,18.67 39,19.93 38.61,20.32 D15.C
  Bottom 0.406: U2.A30 46.35,45.08 | 46.35,45.08 U2.A28 | 46.35,45.08 U2.A29 U2.A31 40.64,40.01 40.64,26.02 34.24,19.62 v34.24,18.67
P1+
  Top 0.406: J8.P$1 J8.P$2 33.92,13.51 33.92,16.13 34.56,16.76 R15.1
P2  (via drill 0.38)
  Top 0.406: v53.18,34.61 51.75,34.61 48.58,31.43 48.58,29.37 v48.26,29.05 | R17.2 48.87,16.69 49.19,17 49.19,18.59 | v43.95,18.59 49.19,18.59 | 49.19,18.59 49.19,19.9 48.77,20.32 D17.C
  Bottom 0.254: U2.A22 56.67,45.08 | 56.67,45.08 U2.A20 | 56.67,43.18 U2.A19 | U2.A21 56.52,44.92 56.67,45.08
  Bottom 0.406: U2.A21 56.67,43.18 56.67,38.1 v53.18,34.61 | v48.26,29.05 49.21,28.1 49.21,24.92 48.85,24.92 43.92,19.99 43.92,18.62 v43.95,18.59
P2+
  Top 0.406: J9.P$1 J9.P$2 46.87,10.48 46.51,10.48 44.13,12.86 44.13,15.92 44.9,16.69 R17.1
P5  (via drill 0.38)
  Top 0.406: v42.86,39.85 40.01,42.7 40.01,43.66 39.69,43.97 39.69,44.61 40.01,44.93 U2.A34 | R19.2 79.5,16.64 79.82,16.95 79.82,18.54 | v75.06,18.54 79.82,18.54 | 79.82,18.54 79.82,20 79.5,20.32 D19.C
  Bottom 0.406: v75.06,18.54 74.74,18.22 74.74,17.11 72.71,15.08 65.88,15.08 65.86,15.06 61.54,15.06 59.94,16.66 59.94,22.17 45.29,36.83 43.5,36.83 42.86,37.47 v42.86,39.85
P5+
  Top 0.406: J10.P$1 J10.P$2 76.75,11.33 R19.1
P8  (via drill 0.38)
  Top 0.406: U2.A27 49.21,42.86 49.21,37.78 46.99,35.56 46.99,32.7 v47.31,32.38 | R7.2 59.05,16.69 59.37,17 59.37,18.59 | v54.61,18.59 59.37,18.59 | 59.37,18.59 59.37,19.88 58.93,20.32 D8.C
  Bottom 0.406: v54.61,18.59 52.7,20.5 52.7,26.99 v47.31,32.38
P8+
  Top 0.406: J11.P$1 J11.P$2 54.45,13.3 54.45,16.05 55.09,16.69 R7.1
P11  (via drill 0.38)
  Top 0.406: v52.7,39.37 58.74,33.34 65.85,33.34 v66.94,32.24 | R9.2 89.41,16.69 89.73,17 89.73,18.59 89.73,18.8 | v85.12,18.75 89.68,18.75 89.73,18.8 | 89.73,18.8 89.73,20 89.41,20.32 D10.C
  Bottom 0.406: U2.A24 v52.7,39.37 | v66.94,32.24 66.95,32.26 69.39,32.26 71.75,29.9 71.75,24.77 73.82,22.7 76.77,22.7 80.72,18.75 v85.12,18.75
P11+
  Top 0.406: J18.P$1 J18.P$2 84.96,13.27 84.96,16.05 85.6,16.69 R9.1
P12
  Top 0.254: D1.4 36.75,26.99 28.74,26.99 28.22,26.47 28.22,25.63 U3.13
P12LL  (via drill 0.38)
  Top 0.254: v47.31,40.32 45.09,38.1 35.56,38.1 31.47,34.01 31.47,31.17 29.97,29.67 28.6,29.67 28.2,30.07 U3.2 | v50.8,40.64 51.44,40.64 U2.A23
  Bottom 0.254: v47.31,40.32 50.48,40.32 v50.8,40.64
P13  (via drill 0.38)
  Top 0.406: v54.93,54.29 12.83,54.29 J12.P$2
  Bottom 0.254: U2.A18 59.38,45.08 57.78,46.67 57.78,47.31 56.52,48.58 56.52,49.21 56.36,49.37 56.36,52.86 v54.93,54.29
  Bottom 0.406: J12.P$1 J12.P$2
P14
  Bottom 0.254: U2.A17 61.59,45.4 62.87,46.67 62.87,47.31 61.59,48.58 61.59,51.75 61.57,51.78 61.57,52.86 57.59,56.83 18.73,56.83 15.24,53.34 15.24,52.38 J13.P$2
  Bottom 0.406: J13.P$1 J13.P$2
P15  (via drill 0.38)
  Top 0.254: U2.A16 61.91,45.09 60.33,46.67 60.33,47.31 59.05,48.58 59.05,49.21 58.74,49.53 58.74,49.85 57.47,51.12 31.43,51.12 v29.84,49.53
  Bottom 0.254: v29.84,49.53 21.27,49.53 21.27,49.52 J14.P$2
  Bottom 0.406: J14.P$1 J14.P$2
P16  (via drill 0.38)
  Top 0.406: R13.2 69.15,16.8 69.41,17.06 69.41,18.64 | v64.48,18.64 69.41,18.64 | 69.41,18.64 69.41,20 69.09,20.32 D13.C
  Bottom 0.406: U2.A15 63.18,42.23 63.18,29.37 62.07,28.26 62.07,19.95 63.35,18.67 64.46,18.67 v64.48,18.64
P16+
  Top 0.406: J15.P$1 J15.P$2 64.64,13.27 64.64,16.26 65.18,16.8 R13.1
P19  (via drill 0.38)
  Top 0.254: U2.A8 73.03,47.31 71.75,48.58 71.75,49.21 69.22,51.75 30.8,51.75 28.57,49.53 v28.57,47.31 | v25.08,47.31 15.24,37.47 15.24,34.6 J16.P$2
  Top 0.406: J16.P$1 J16.P$2
  Bottom 0.254: v28.57,47.31 v25.08,47.31
P20  (via drill 0.38)
  Top 0.254: v25.4,50.48 26.67,49.21 26.67,46.04 20.64,40.01 20.64,35.56 14.29,29.21 14.29,24.77 J17.P$2 | v63.5,50.8 63.82,51.12 67.31,51.12 69.22,49.21 69.22,48.58 70.48,47.31 70.48,46.67 71.75,45.4 71.75,44.77 73.34,43.18 U2.A7 | v25.4,55.24 25.4,58.74 27.3,60.64 61.59,60.64 63.34,58.9 v63.34,56.52
  Bottom 0.254: v25.4,50.48 v25.4,55.24 | v63.34,56.52 63.34,50.96 v63.5,50.8
  Bottom 0.406: J17.P$1 9.78,21.02 10.16,20.64 10.17,20.64 J17.P$2
PD
  Top 0.406: S3.1 19.36,6.99 20.32,6.99 20.8,7.46 20.8,15.88 23.62,18.69 28.92,18.69 | R11.2 28.6,16.79 28.92,17.11 28.92,18.69 | 28.92,18.69 28.92,19.05 28.92,19.85 28.45,20.32 D12.C
V_BATT
  Top 0.305: D14.A 92.71,10.16 93.93,8.94 J19.PWR
VIN  (via drill 0.38)
  Top 0.254: 86.74,31.76 86.91,31.93 | C13.1 79.26,33.68 78.61,34.33 78.61,36.83 78.61,36.84 78.61,36.89 | 77.53,36.89 78.61,36.89 | 78.61,36.89 D7.A
  Top 0.305: D6.C 93.98,17.66 | 93.98,17.66 D14.C | 93.98,17.66 93.98,19.81 90.93,22.86 87.88,22.86 85.47,25.27 85.47,27.56
  Top 0.406: D16.C 77.53,36.89
  other vias: 80.07,32.26 80.07,31.24 80.14,30.26 80.11,29.31 80.11,28.29 83.6,32.16
  pour Top (isolate 0.305): 79.34,34.23 84.68,34.32 84.71,32.48 84.93,32.48 87,32.51 87,31.59 86.04,31.59 85.57,31.11 85.57,26.99 79.34,26.92
  pour Bottom (isolate 0.305): 79.33,34.26 84.68,34.35 84.68,32.51 87,32.51 87,31.75 85.5,31.73 85.61,26.95 79.26,26.92
VIN_TAB
  Top 0.305: J3.P$2 98.48,21.02 97.79,20.32 97.79,16.51 96.64,15.36 D6.A
  Top 0.406: J3.P$2 J3.P$1
VOUT3.3
  Top 0.254: J6.P$2 J6.P$1
  Top 0.406: S1.3 94.89,52.4 95.66,53.16 97.79,53.16 | 97.79,53.16 100.35,53.16 J6.P$2 | D9.A 97.71,53.24 97.79,53.16
VOUT5.0
  Top 0.406: S1.6 94.89,37.92 96.01,36.8 97.61,36.8 | J1.P$1 J1.P$2 101.83,36.8 97.61,36.8 | D11.A 97.62,38.02 97.62,36.82 97.61,36.8

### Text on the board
Bottom: v20
Measures: * All dimensions / are in inches
tDocu: Mary West | Andy England | Solder Mask: Black Gloss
